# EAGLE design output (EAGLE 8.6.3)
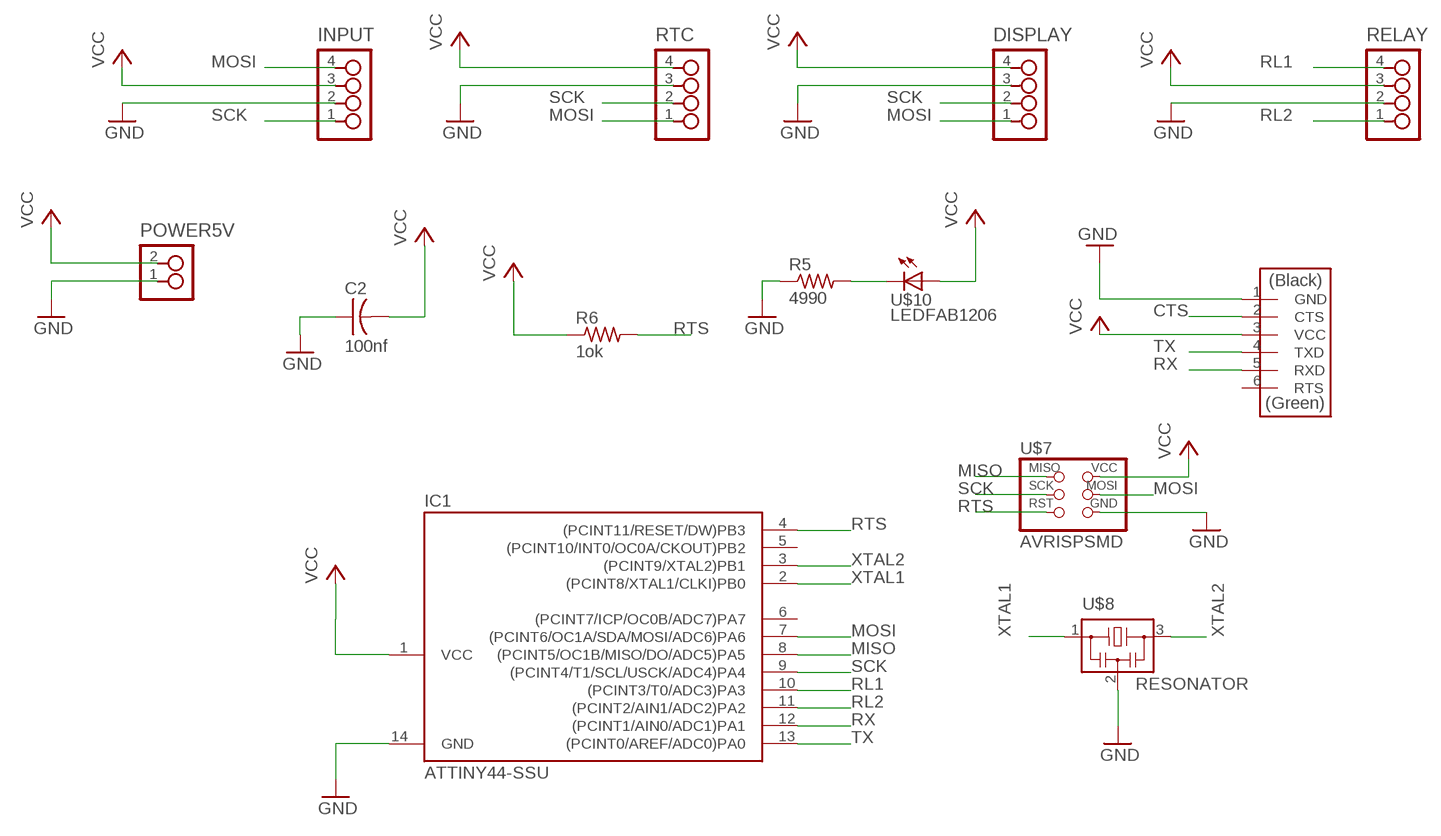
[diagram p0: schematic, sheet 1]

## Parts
C2  100nf  CAP-US1206K  [C1206K]
DISPLAY  4_PIN_HEADERHEADER  [SMT_PINS_4]
FTDI  FTDI-SMD-HEADER  [1X06SMD]
IC1  ATTINY44-SSU  [SOIC14]
INPUT  4_PIN_HEADERHEADER  [SMT_PINS_4]
POWER5V  2_PIN_HEADERHEADER  [SMT_PINS_2]
R5  4990  RES-US1206FAB  [R1206FAB]
R6  1ok  RES-US1206FAB  [R1206FAB]
RELAY  4_PIN_HEADERHEADER  [SMT_PINS_4]
RTC  4_PIN_HEADERHEADER  [SMT_PINS_4]
U$7  AVRISPSMD  [2X03SMD]
U$8  RESONATOR  [EFOBM]
U$10  LEDFAB1206  [LED1206FAB]

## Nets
CTS: FTDI.2(CTS)
GND: C2.1 DISPLAY.3 FTDI.1(GND) IC1.14(GND) INPUT.2 POWER5V.1 R5.1 RELAY.2 RTC.3 U$7.6(GND) U$8.2
MISO: IC1.8((PCINT5/OC1B/MISO/DO/ADC5)PA5) U$7.1(MISO)
MOSI: DISPLAY.1 IC1.7((PCINT6/OC1A/SDA/MOSI/ADC6)PA6) INPUT.4 RTC.1 U$7.4(MOSI)
N$7: R5.2 U$10.2(C)
RL1: IC1.10((PCINT3/T0/ADC3)PA3) RELAY.4
RL2: IC1.11((PCINT2/AIN1/ADC2)PA2) RELAY.1
RTS: IC1.4((PCINT11/RESET/DW)PB3) R6.2 U$7.5(RST)
RX: FTDI.5(RXD) IC1.12((PCINT1/AIN0/ADC1)PA1)
SCK: DISPLAY.2 IC1.9((PCINT4/T1/SCL/USCK/ADC4)PA4) INPUT.1 RTC.2 U$7.3(SCK)
TX: FTDI.4(TXD) IC1.13((PCINT0/AREF/ADC0)PA0)
VCC: C2.2 DISPLAY.4 FTDI.3(VCC) IC1.1(VCC) INPUT.3 POWER5V.2 R6.1 RELAY.3 RTC.4 U$7.2(VCC) U$10.1(A)
XTAL1: IC1.2((PCINT8/XTAL1/CLKI)PB0) U$8.1
XTAL2: IC1.3((PCINT9/XTAL2)PB1) U$8.3
Unconnected: FTDI.6(RTS) IC1.5((PCINT10/INT0/OC0A/CKOUT)PB2) IC1.6((PCINT7/ICP/OC0B/ADC7)PA7)

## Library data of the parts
C2 = fab:CAP-US
DISPLAY INPUT RELAY RTC = FabLab:4_PIN_HEADER: 4 SMT pin pads
FTDI = fab:FTDI-SMD-HEADER
IC1 = fab:ATTINY44
POWER5V = FabLab:2_PIN_HEADER: 2 SMT pin pads
R5 R6 = fab:RES-US: Resistor (US Symbol)
U$7 = fab:AVRISP
U$8 = fab:RESONATOR
U$10 = fab:LED: LED

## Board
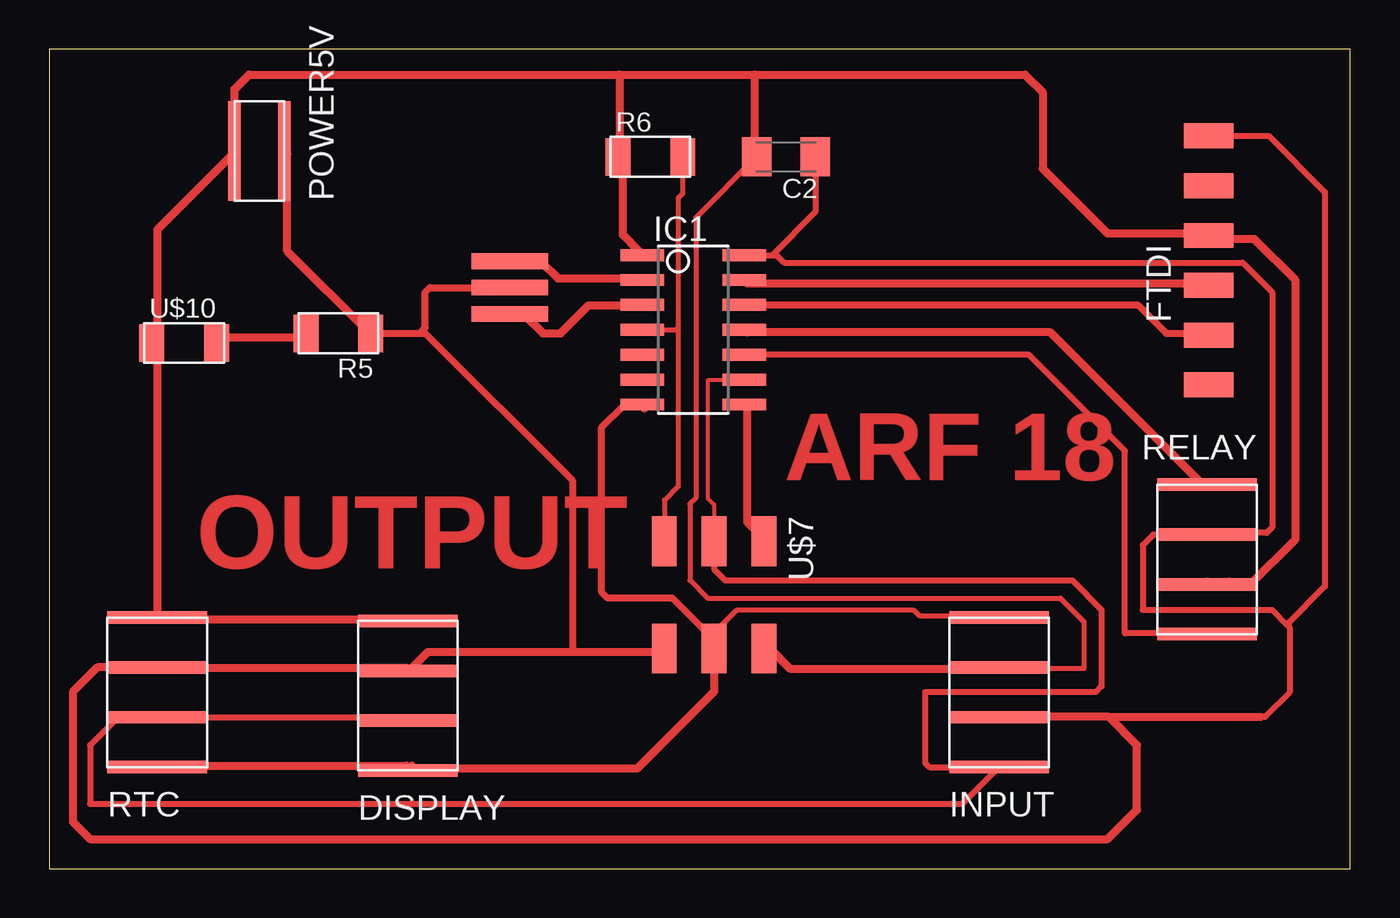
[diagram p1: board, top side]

Size 66.4 x 41.8 mm. Coordinates in mm from the lower left corner, seen from the top.
Outline: 0,0 66.4,0 66.4,41.8 0,41.8 0,0
Copper layers (1*16): Top 0.035mm / dielectric 1.5mm / Bottom 0.035mm
Design rules "default *": minimum track width 0.4mm, minimum drill 0.35mm, track to track 6mil, track to pad 6mil, pad to pad 6mil, via to via 6mil, smd to smd 6mil, copper to edge 40mil, drill to drill 6mil, minimum pad ring 10mil, minimum via ring 8mil, stop-mask expansion 4mil, vias tented up to drill 0mil, thermal gap 10mil

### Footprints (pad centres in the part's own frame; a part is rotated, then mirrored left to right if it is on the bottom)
C1206K = smd 1.5 x 2: 1 -1.5,0; 2 1.5,0
SMT_PINS_4 = smd 5.08 x 0.635: 1 0,0; 2 0,2.54; 3 0,5.08; 4 0,7.62
1X06SMD = smd 2.54 x 1.27: 1 0,6.35; 2 0,3.81; 3 0,1.27; 4 0,-1.27; 5 0,-3.81; 6 0,-6.35
SOIC14 = smd 0.61 x 2.21: 1 -3.81,-2.603; 2 -2.54,-2.603; 3 -1.27,-2.603; 4 0,-2.603; 5 1.27,-2.603; 6 2.54,-2.603; 7 3.81,-2.603; 8 3.81,2.603; 9 2.54,2.603; 10 1.27,2.603; 11 0,2.603; 12 -1.27,2.603; 13 -2.54,2.603; 14 -3.81,2.603
SMT_PINS_2 = smd 5.08 x 0.635: 1 0,0; 2 0,2.54
R1206FAB = smd 1.27 x 1.905: 1 -1.651,0; 2 1.651,0
2X03SMD = smd 2.54 x 1.27: 1 -2.54,2.54; 2 2.92,2.54; 3 -2.54,0; 4 2.92,0; 5 -2.54,-2.54; 6 2.92,-2.54
EFOBM = smd 0.8 x 3.9: 1 -1.35,0; 2 0,0; 3 1.35,0
LED1206FAB = smd 1.27 x 1.905: 1 -1.651,0; 2 1.651,0

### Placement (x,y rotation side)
C2  37.6,36.3 180 top
DISPLAY  18.3,5.01 0 top
FTDI  59.16,31.02 0 top
IC1  32.87,27.48 270 top
INPUT  48.47,5.18 0 top
POWER5V  12,36.6 90 top
R5  14.76,27.3 180 top
R6  30.68,36.3 0 top
RELAY  59.09,19.58 180 top
RTC  5.52,5.18 0 top
U$7  33.93,14.15 270 top
U$8  23.52,29.63 270 top
U$10  6.9,26.81 0 top

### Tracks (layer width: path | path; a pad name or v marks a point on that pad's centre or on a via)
GND
  Top 0.305: IC1.14 36.9,31.29 | 36.9,31.29 37.11,31.29 37.5,30.9 60.9,30.9 62.4,29.4 62.4,17.4 62.12,17.12 59.4,17.12 | RELAY.2 56.34,17.04 55.8,16.5 55.8,13.2 62.4,13.2 63.15,12.45 | 63.15,12.45 63.3,12.3 63.3,9 62.03,7.73 61.8,7.73 | FTDI.1 62.23,37.37 65.1,34.5 65.1,14.4 63.15,12.45 | C2.1 39.1,33.49 36.9,31.29
  Top 0.35: R5.1 18.9,27.3 | 18.9,27.3 19.2,27.3 26.7,19.8 26.7,11.05 | 18.9,27.3 19.2,27.6 19.2,29.4 19.43,29.63 U$8.2
  Top 0.4: 59.38,37.29 FTDI.1 | 60.21,17.12 59.4,17.12 59.11,17.12 RELAY.2 | INPUT.2 48.61,7.73 54.07,7.73 | 16.57,27.34 R5.1 16.3,27.34 12.15,31.49 12.15,36.46 POWER5V.1 | U$7.6 31.21,11.05 26.7,11.05 19.33,11.05 18.5,10.22 DISPLAY.3 18.23,10.22 5.52,10.22 RTC.3 | 4.42,10.22 5.25,10.22 RTC.3 | RTC.3 2.46,10.26 1.22,9.02 1.22,2.38 2.1,1.5 54,1.5 55.5,3 55.5,6.3 54.07,7.73 | 54.07,7.73 61.8,7.73
MISO
  Top 0.4: IC1.8 35.63,23.48 35.63,17.68 36.46,16.85 U$7.1
MOSI
  Top 0.254: 48.37,12.9 44.4,12.9 44.1,13.2 35.1,13.2 33.93,12.03
  Top 0.305: U$7.4 33.93,12.03 | 48.37,12.9 INPUT.4
  Top 0.35: U$7.4 33.93,11.67 31.8,13.8 28.5,13.8 28.2,14.1 28.2,22.5 29.37,23.67 IC1.7
  Top 0.4: DISPLAY.1 18.23,5.25 5.52,5.25 RTC.1 | 30.38,23.48 IC1.7 | 33.97,11.32 U$7.4 | 18.5,5.25 DISPLAY.1 | 33.7,11.05 U$7.4 | U$7.4 33.93,9.03 30,5.1 18.39,5.1 DISPLAY.1
N$7
  Top 0.4: U$10.2 8.56,27.07 12.98,27.07 R5.2
RL1
  Top 0.305: 59.05,12 54.9,12 54.9,21.3 49.99,26.21 IC1.10
  Top 0.4: RELAY.4 59.05,12
RL2
  Top 0.4: IC1.11 35.63,27.34 51.1,27.34 58.83,19.61 RELAY.1
RTS
  Top 0.254: R6.2 32.33,34.43 32.1,34.2 32.1,27.6 | 30.45,27.3 IC1.4 31.98,27.48 32.1,27.6 | 32.1,27.6 32.1,19.5 31.39,18.79 U$7.5
  Top 0.4: 31.49,16.85 U$7.5
RX
  Top 0.35: IC1.12 55.55,28.75 57,27.3 59.07,27.3 FTDI.5
  Top 0.4: 35.63,28.73 IC1.12 | 59.11,27.34 FTDI.5
SCK
  Top 0.203: IC1.9 35.43,24.9 33.6,24.9 33.6,18.9 33.93,18.57 33.93,16.5
  Top 0.254: 33.9,16.72 U$7.3
  Top 0.305: 3.52,7.72 2.1,6.3 2.1,3.3 46.59,3.3 INPUT.1 44.92,5.18 44.7,5.4 44.7,9 53.4,9 53.7,9.3 53.7,13.2 52.2,14.7 34.5,14.7 33.93,15.27 33.93,16.5 U$7.3 | RTC.2 18.13,7.72 DISPLAY.2
  Top 0.4: 5.52,7.73 RTC.2 3.52,7.72
TX
  Top 0.4: IC1.13 35.63,29.83 59.11,29.83 FTDI.4
VCC
  Top 0.254: INPUT.3 48.53,10.2 52.8,10.2 52.8,12.6 51.6,13.8 33.6,13.8 32.7,14.7 32.7,18.6 33,18.9 33,33.2 C2.2
  Top 0.4: 60.21,32.04 59.7,32.04 | 59.7,32.04 59.38,32.04 FTDI.3 | 60.21,14.64 59.11,14.64 RELAY.3 61.3,14.5 63.6,16.8 63.6,30 61.5,32.1 59.35,32.1 FTDI.3 | DISPLAY.4 18.23,12.71 5.52,12.71 RTC.4 5.52,12.98 5.52,26.79 U$10.1 5.52,27.07 5.52,32.59 9.39,36.46 POWER5V.2 9.46,39.76 10.2,40.5 29.1,40.5 | R6.1 29.28,36.18 29.28,32.31 30.11,31.49 IC1.1 | 35.91,36.46 C2.2 36,36.4 36,40.5 | 29.28,36.46 R6.1 | R6.1 29,36.46 29.1,36.56 29.1,40.5 | 59.11,32.31 FTDI.3 | 29.1,40.5 36,40.5 | 36,40.5 49.8,40.5 50.7,39.6 50.7,35.7 54,32.4 59.34,32.4 59.7,32.04 | U$7.2 36.77,11.23 37.8,10.2 48.41,10.2 INPUT.3
XTAL1
  Top 0.4: IC1.2 30.11,30.11 25.96,30.11 25.13,30.93 23.75,30.93 U$8.1
XTAL2
  Top 0.4: 30.11,28.73 IC1.3 | 23.75,28.45 U$8.3
  Top 0.406: U$8.3 24.22,28.28 25.2,27.3 26.1,27.3 27.52,28.73 30.11,28.73

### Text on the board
Top: ARF 18 | OUTPUT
